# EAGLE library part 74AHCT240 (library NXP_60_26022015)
Octal buffer/line driver; inverting; 3-state The 74AHC240 and 74AHCT240 are 8-bit inverting buffer/line drivers with 3-state outputs. These devices can be used as two 4-bit buffers or one 8-bit buffer. They feature two output enables (1OE and 2OE), each controlling four of the 3-state outputs. A HIGH on nOE causes the outputs to assume a high-impedance OFF-state. Inputs are over voltage tolerant. This feature allows the use of these devices as translators in mixed voltage environments. AAL Eindhoven MK
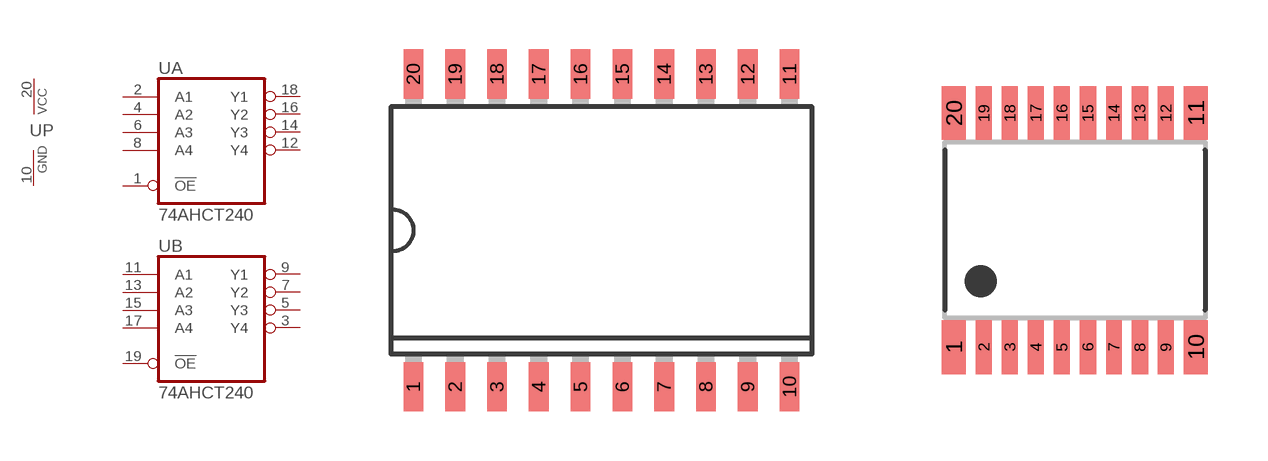
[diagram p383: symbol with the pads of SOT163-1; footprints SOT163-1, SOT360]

Designator prefix U; gates A=74240 B=74240 P=PWRN-3

## 74AHCT240D  [SOT163-1]
1  A:!OE  in
2  A:A1  in
3  B:Y4  hiz
4  A:A2  in
5  B:Y3  hiz
6  A:A3  in
7  B:Y2  hiz
8  A:A4  in
9  B:Y1  hiz
10  P:GND  pwr
11  B:A1  in
12  A:Y4  hiz
13  B:A2  in
14  A:Y3  hiz
15  B:A3  in
16  A:Y2  hiz
17  B:A4  in
18  A:Y1  hiz
19  B:!OE  in
20  P:VCC  pwr

## 74AHCT240PW  [SOT360]
Pads as for SOT163-1

## 74AHCT240BQ  [SOT764]
1  A:!OE  in
2  A:A1  in
3  B:Y4  hiz
4  A:A2  in
5  B:Y3  hiz
6  A:A3  in
7  B:Y2  hiz
8  A:A4  in
9  B:Y1  hiz
10  P:GND  pwr
11  B:A1  in
12  A:Y4  hiz
13  B:A2  in
14  A:Y3  hiz
15  B:A3  in
16  A:Y2  hiz
17  B:A4  in
18  A:Y1  hiz
19  B:!OE  in
20  P:VCC  pwr
CP  P:GND  pwr

## Footprint SOT163-1 (pad centres in mm)
SOT163-1 SO20: plastic small outline package; 20 leads; body width 7.5 mm JEDEC: MS-013 IEC: 075E04
smd 0.6 x 1.5: 1 -5.715,-4.75; 2 -4.445,-4.75; 3 -3.175,-4.75; 4 -1.905,-4.75; 5 -0.635,-4.75; 6 0.635,-4.75; 7 1.905,-4.75; 8 3.175,-4.75; 9 4.445,-4.75; 10 5.715,-4.75; 11 5.715,4.75; 12 4.445,4.75; 13 3.175,4.75; 14 1.905,4.75; 15 0.635,4.75; 16 -0.635,4.75; 17 -1.905,4.75; 18 -3.175,4.75; 19 -4.445,4.75; 20 -5.715,4.75

## Footprint SOT360 (pad centres in mm)
SOT360 TSSOP20: plastic thin shrink small outline package; 20 leads; body width 4.4 mm JEDEC: MO-153 IEC:
smd 0.6 x 1.35: 1 -3.025,-2.925; 10 3.025,-2.925; 11 3.025,2.925; 20 -3.025,2.925
smd 0.4 x 1.35: 2 -2.275,-2.925; 3 -1.625,-2.925; 4 -0.975,-2.925; 5 -0.325,-2.925; 6 0.325,-2.925; 7 0.975,-2.925; 8 1.625,-2.925; 9 2.275,-2.925; 12 2.275,2.925; 13 1.625,2.925; 14 0.975,2.925; 15 0.325,2.925; 16 -0.325,2.925; 17 -0.975,2.925; 18 -1.625,2.925; 19 -2.275,2.925

## Footprint SOT764 (pad centres in mm)
SOT764 DHVQFN20: plastic dual in-line compatible thermal enhanced very thin quad flat package; no leads; 20 terminals; body 2.5 x 4.5 x 0.85 mm JEDEC: MO-241 IEC: ---
smd 1 x 0.29: 1 -2.25,-0.25; 10 2.25,-0.25; 11 2.25,0.25; 20 -2.25,0.25
smd 0.29 x 1: 2 -1.75,-1.35; 3 -1.25,-1.35; 4 -0.75,-1.35; 5 -0.25,-1.35; 6 0.25,-1.35; 7 0.75,-1.35; 8 1.25,-1.35; 9 1.75,-1.35; 12 1.75,1.35; 13 1.25,1.35; 14 0.75,1.35; 15 0.25,1.35; 16 -0.25,1.35; 17 -0.75,1.35; 18 -1.25,1.35; 19 -1.75,1.35
smd 2.9 x 0.9: CP 0,0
